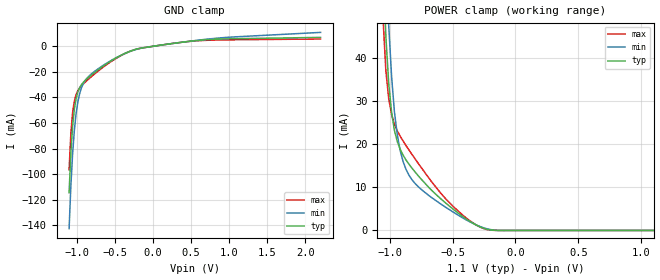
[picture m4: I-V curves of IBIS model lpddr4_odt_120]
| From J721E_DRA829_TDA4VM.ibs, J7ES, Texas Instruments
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|1LPDDR4 ********** Begin LPDDR4 Models
|   Model lpddr4_odt_120
[Model] lpddr4_odt_120
Model_type Input
Polarity   Non-Inverting
Enable   Active-High
Vinl =  0.0V
Vinh =  0.900V
C_comp   2.469pF   2.415pF   2.634pF
[Model Spec]
Vinh   0.900V   0.900V   0.900V
Vinl   0.0V   0.0V   0.0V
[Temperature Range]   25.000   0.125k   -40.000
[Voltage Range]   1.100V   1.060V   1.170V
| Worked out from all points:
|   GND clamp passes 1 mA (typ) near -0.11 V on its own axis
|   POWER clamp passes 1 mA (typ) near -0.29 V on its own axis
[GND_clamp]
|Voltage   I(typ)   I(min)   I(max)
-1.1V     -114.5mA   -142.6mA   -96.6mA
-1.077V   -83.44mA   -109.3mA   -68.41mA
-1.054V   -62.46mA   -84.08mA   -51.87mA
-1.031V   -49.11mA   -65.64mA   -42.78mA
-1.008V   -40.88mA   -52.58mA   -37.76mA
-985mV    -35.77mA   -43.5mA    -34.75mA
-917mV    -28.43mA   -29.61mA   -29.64mA
-779mV    -21.16mA   -20.23mA   -22.32mA
-390mV    -6.16mA    -6.305mA   -6.361mA
-115mV    -1.046mA   -1.079mA   -1.085mA
642mV     4.827mA    5.103mA    4.501mA
2.2V      6.95mA     10.85mA    5.7mA
[POWER_clamp]
|Voltage   I(typ)   I(min)   I(max)
-1.1V     137.1mA    171.2mA    113.1mA
-1.054V   63.77mA    90.19mA    49.8mA
-1.031V   45.29mA    65.16mA    37.27mA
-1.008V   34.15mA    47.69mA    30.66mA
-963mV    23.33mA    27.72mA    24.77mA
-940mV    20.69mA    22.28mA    23.17mA
-894mV    17.53mA    16.05mA    20.82mA
-848mV    15.46mA    12.91mA    18.77mA
-665mV    9.284mA    7.606mA    11.25mA
-435mV    3.583mA    3.189mA    3.97mA
-229mV    284.6uA    401.3uA    226.1uA
1.1V      0A         0A         0A
